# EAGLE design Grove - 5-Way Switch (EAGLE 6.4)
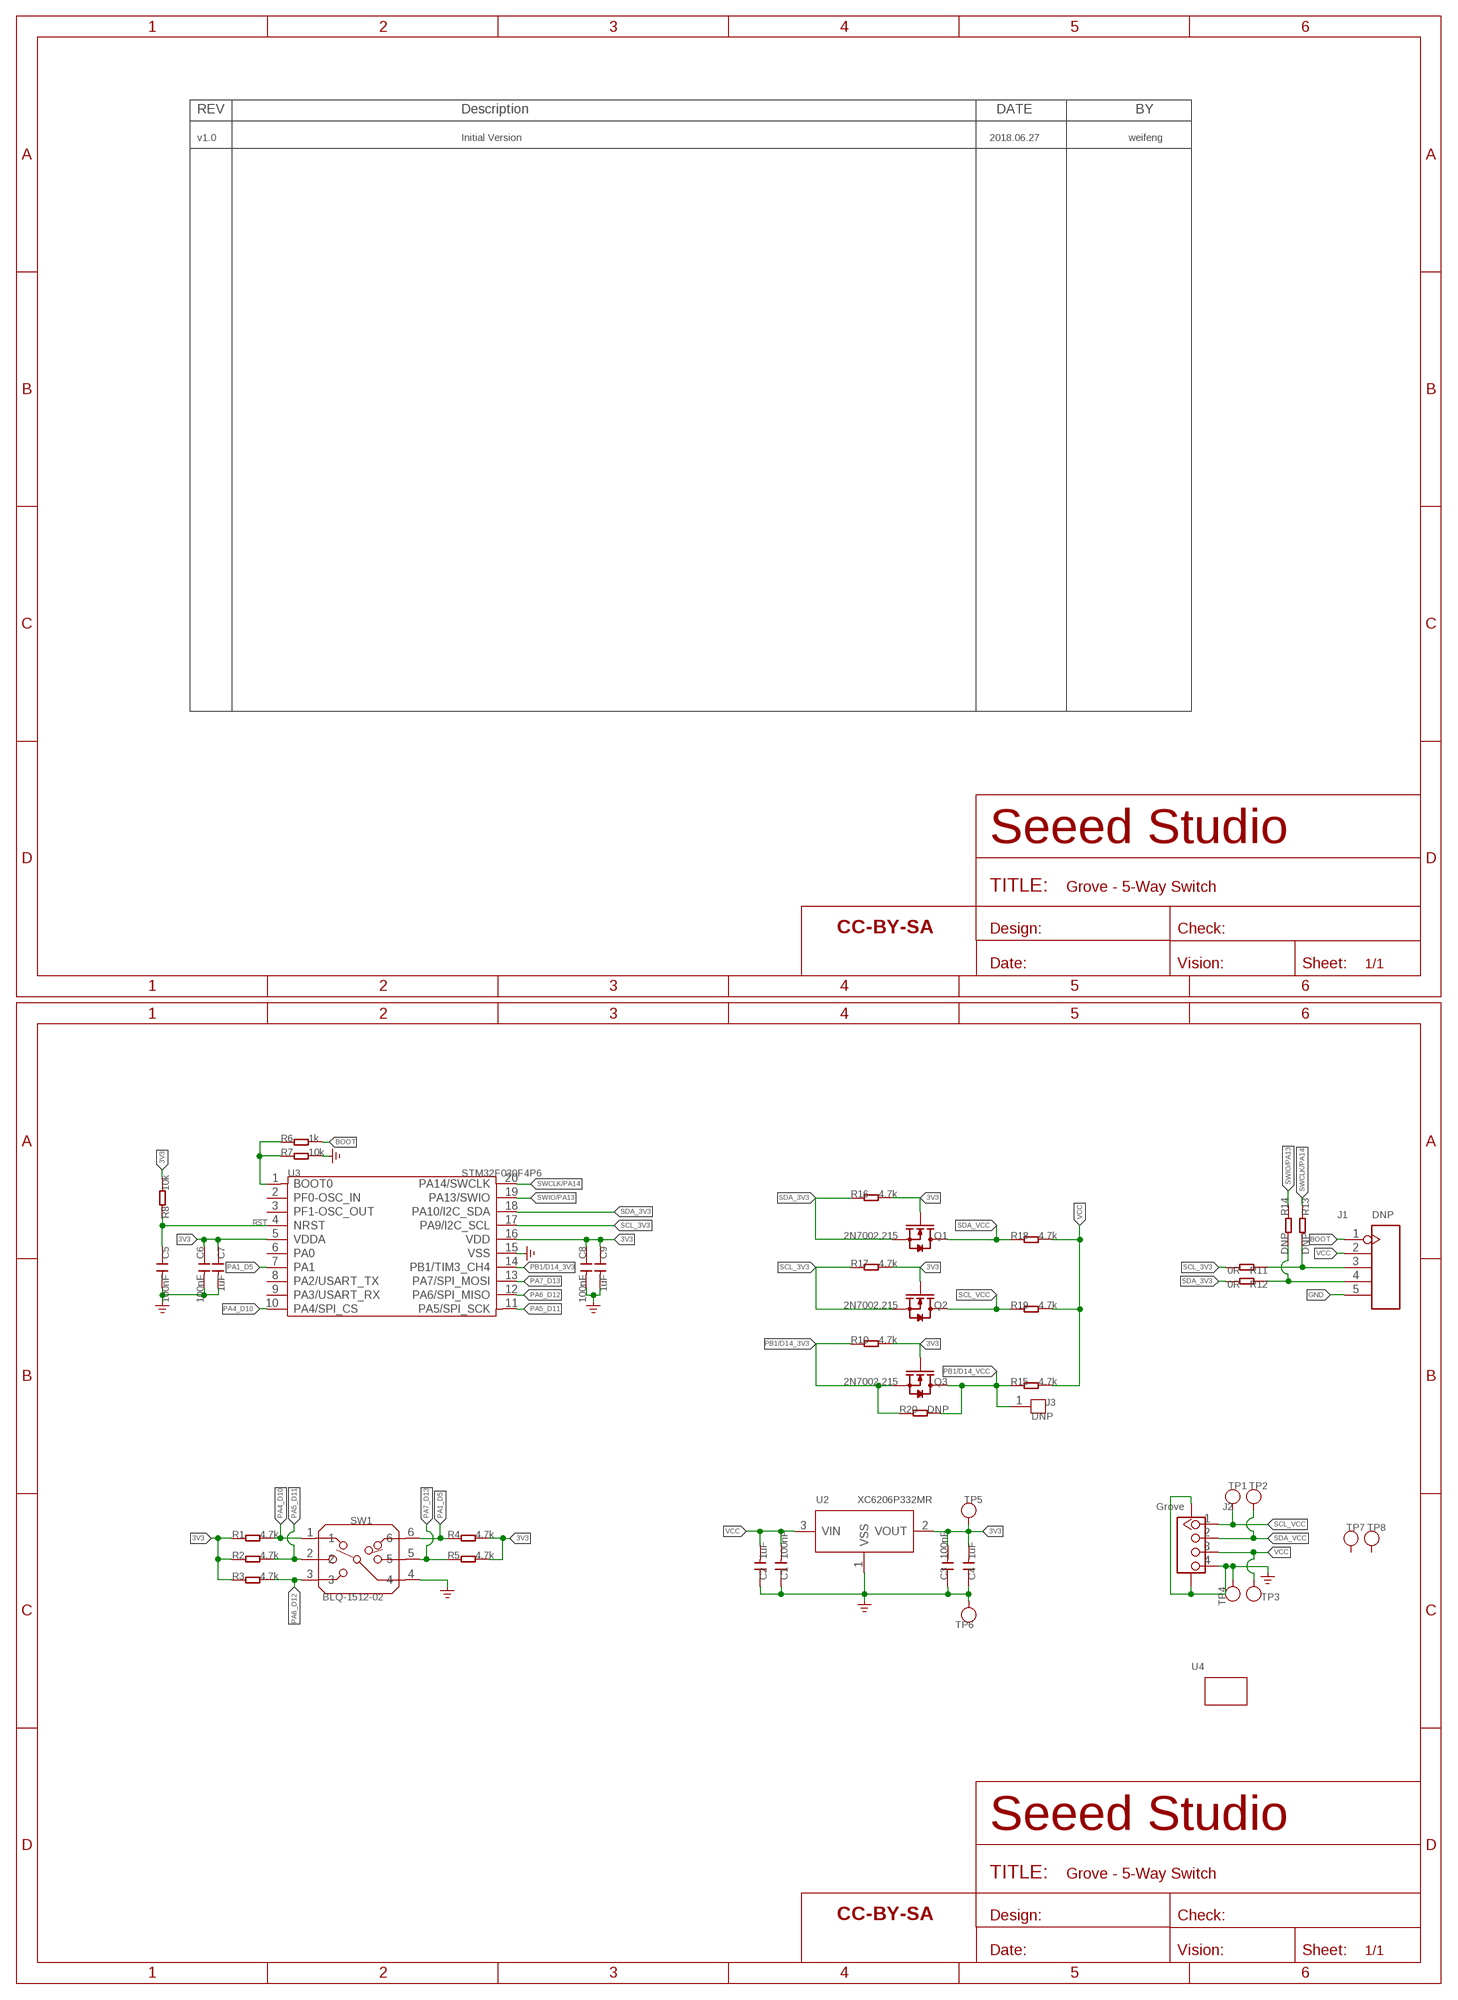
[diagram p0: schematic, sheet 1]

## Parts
C1  100nF  C-0603  [C0603]
C2  1uF  C-0603  [C0603]
C3  100nF  C-0603  [C0603]
C4  1uF  C-0603  [C0603]
C5  100nF  C-0603  [C0603]
C6  100nF  C-0603  [C0603]
C7  1uF  C-0603  [C0603]
C8  100nF  C-0603  [C0603]
C9  1uF  C-0603  [C0603]
FR1  SEEEDSTUDIO-OPEN-SCH-FRAME  [SEEEDSTUDIO-PCB-FRAME]
J1  DNP  HEADER-5P-SMD2.54  [H5-SMD-2.54]
J2  Grove  GROVE-CONNECTOR-SMD'DD'  [HW4-SMD-2.0]
J3  DNP  HEADER-1P-35  [1P-65/35MIL]
Q1  2N7002,215  MOSFET-N'SOT23'  [SOT-23]
Q2  2N7002,215  MOSFET-N'SOT23'  [SOT-23]
Q3  2N7002,215  MOSFET-N'SOT23'  [SOT-23]
R1  4.7k  R-0603  [R0603]
R2  4.7k  R-0603  [R0603]
R3  4.7k  R-0603  [R0603]
R4  4.7k  R-0603  [R0603]
R5  4.7k  R-0603  [R0603]
R6  1k  R-0603  [R0603]
R7  10k  R-0603  [R0603]
R8  10k  R-0603  [R0603]
R10  4.7k  R-0603  [R0603]
R11  0R  R-0603  [R0603]
R12  0R  R-0603  [R0603]
R13  DNP  R-0603  [R0603]
R14  DNP  R-0603  [R0603]
R15  4.7k  R-0603  [R0603]
R16  4.7k  R-0603  [R0603]
R17  4.7k  R-0603  [R0603]
R18  4.7k  R-0603  [R0603]
R19  4.7k  R-0603  [R0603]
R20  DNP  R-0603  [R0603]
SW1  BLQ-1512-02  SWITCH-6P  [SW6-3.25-10.2X10.2X6MM]
TP1  TEST-POINT'4545'  [TP-D45MIL]
TP2  TEST-POINT'4545'  [TP-D45MIL]
TP3  TEST-POINT'4545'  [TP-D45MIL]
TP4  TEST-POINT'4545'  [TP-D45MIL]
TP5  TEST-POINT'4545'  [TP-D45MIL]
TP6  TEST-POINT'4545'  [TP-D45MIL]
TP7  TEST-POINT'4545'  [TP-D45MIL]
TP8  TEST-POINT'4545'  [TP-D45MIL]
U2  XC6206P332MR  PMIC-XC6206PMR  [SOT-23]
U3  STM32F030F4P6  MCU-STM32F030  [TSSOP20-0.65-6.5X4.4MM]
U4  GROVE-TOP  [GROVE-1*2-TEST-PLATFORM-TOP]
U$4  SEEEDSTUDIO-OPEN-SCH-FRAME  [SEEEDSTUDIO-PCB-FRAME]

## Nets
3V3: C3.2 C4.2 C6.1 C7.1 C8.1 C9.1 Q1.1(G) Q2.1(G) Q3.1(G) R1.1 R2.1 R3.1 R4.2 R5.2 R8.2 R10.2 R16.2 R17.2 TP5.T U2.2(VOUT) U3.5(VDDA) U3.16(VDD)
!RST: C5.1 R8.1 U3.4(NRST)
BOOT: J1.1 R6.2
GND: C1.1 C2.1 C3.1 C4.1 C5.2 C6.2 C7.2 C8.2 C9.2 J1.5 J2.4 J2.SS1 J2.SS2 R7.2 SW1.4 TP4.T TP6.T U2.1(VSS) U3.15(VSS) ; supply symbol labelled GND_POWER
N$1: R6.1 R7.1 U3.1(BOOT0)
N$3: J1.3 R11.1 R13.2
N$4: J1.4 R12.1 R14.2
PA1_D5: R4.1 SW1.6 U3.7(PA1)
PA4_D10: R1.2 SW1.1 U3.10(PA4/SPI_CS)
PA5_D11: R2.2 SW1.2 U3.11(PA5/SPI_SCK)
PA6_D12: R3.2 SW1.3 U3.12(PA6/SPI_MISO)
PA7_D13: R5.1 SW1.5 U3.13(PA7/SPI_MOSI)
PB1/D14_3V3: Q3.2(S) R10.1 R20.1 U3.14(PB1/TIM3_CH4)
PB1/D14_VCC: J3.1 Q3.3(D) R15.1 R20.2
SCL_3V3: Q2.2(S) R11.2 R17.1 U3.17(PA9/I2C_SCL)
SCL_VCC: J2.1 Q2.3(D) R19.1 TP1.T
SDA_3V3: Q1.2(S) R12.2 R16.1 U3.18(PA10/I2C_SDA)
SDA_VCC: J2.2 Q1.3(D) R18.1 TP2.T
SWCLK/PA14: R13.1 U3.20(PA14/SWCLK)
SWIO/PA13: R14.1 U3.19(PA13/SWIO)
VCC: C1.2 C2.2 J1.2 J2.3 R15.2 R18.2 R19.2 TP3.T U2.3(VIN)
Unconnected: TP7.T TP8.T U3.2(PF0-OSC_IN) U3.3(PF1-OSC_OUT) U3.6(PA0) U3.8(PA2/USART_TX) U3.9(PA3/USART_RX)

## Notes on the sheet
- v1.0 | Initial Version | 2018.06.27 | weifeng

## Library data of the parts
C1-C9 = Discrete-small:C*: Ceramic Capacitors
FR1 U$4 = moudle-new:SEEEDSTUDIO-OPEN-SCH-FRAME
J1 = Connector-new:HEADER-5P
J2 = Connector-new:GROVE-CONNECTOR-SMD: 4P-SMD-2.0:320110030;4P-SMD-2.0-90D:320110032
J3 = Connector-new:HEADER-1P
Q1-Q3 = Discrete-new:MOSFET-N
R1-R8 R10-R20 = Discrete-small:R*
SW1 = Discrete-new:SWITCH-6P
TP1-TP8 = Discrete-new:TEST-POINT; PARTNO: DNP
U2 = IC-new:PMIC-XC6206P: LOW ESR Cap.Compatible Positive Voltage Regulators
U3 = IC-new:MCU-STM32F030
U4 = moudle-new:GROVE

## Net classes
3 usbvcc: width 0.203 mm, drill 0.305 mm, clearance 0.203 mm

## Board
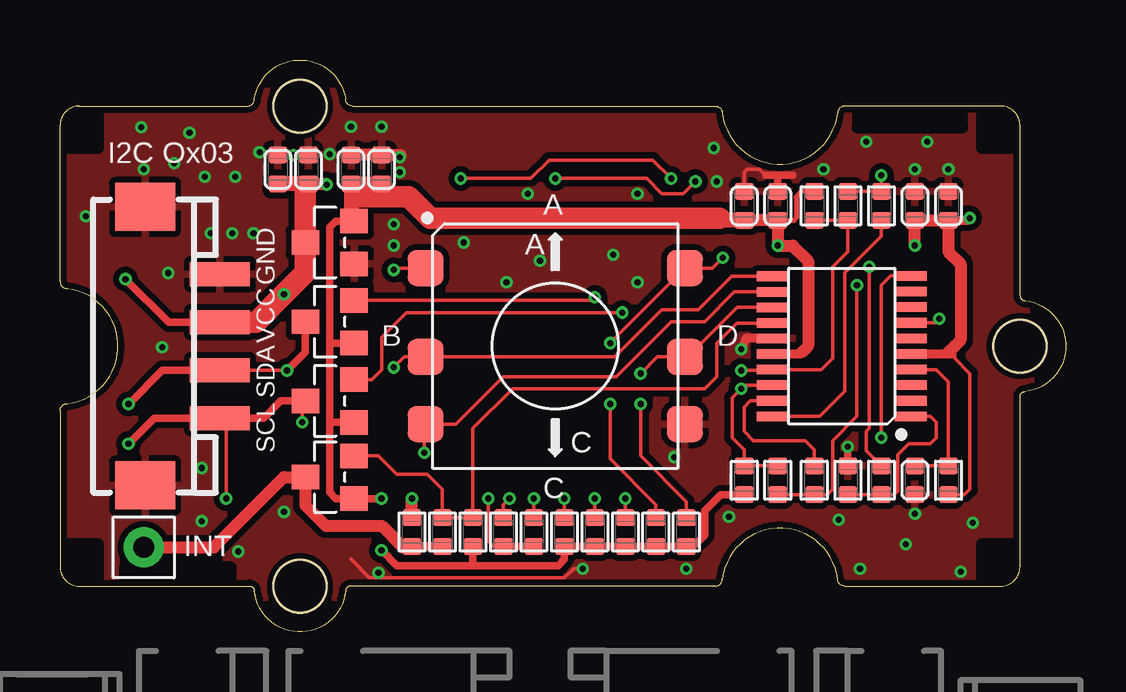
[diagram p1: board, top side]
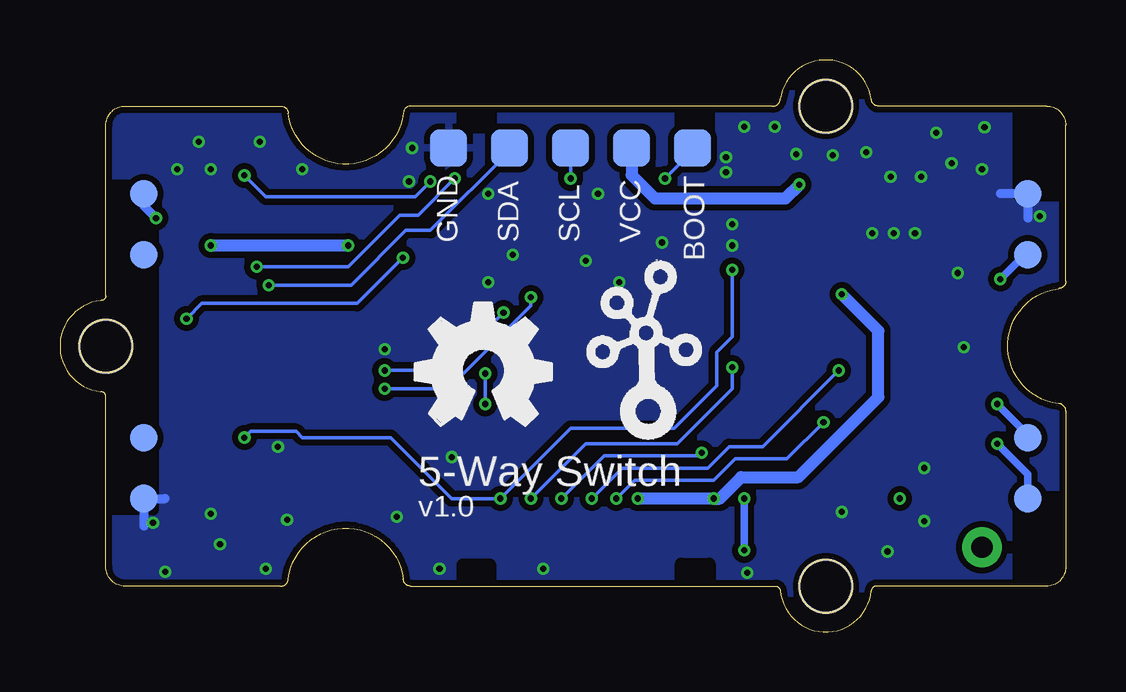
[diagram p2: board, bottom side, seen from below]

Size 41.91 x 23.83 mm. Coordinates in mm from the lower left corner, seen from the top.
Copper layers (1*16): Top 0.035mm / dielectric 1.5mm / Bottom 0.035mm
Design rules "SeeedStudio_2layer_DRU_no_angle_20140221": minimum track width 1mil, minimum drill 10mil, track to track 6mil, track to pad 6mil, pad to pad 6mil, via to via 6mil, smd to smd 0mil, copper to edge 10mil, drill to drill 10mil, minimum pad ring 4mil, minimum via ring 4mil, stop-mask expansion 2mil, vias tented up to drill 25mil, thermal gap 10mil

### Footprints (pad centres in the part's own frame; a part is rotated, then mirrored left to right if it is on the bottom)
C0603 = smd 0.762 x 0.696: 1 0,0.602; 2 0,-0.602
H5-SMD-2.54 = smd 1.524 x 1.524: 1 0,5.08; 2 0,2.54; 3 0,0; 4 0,-2.54; 5 0,-5.08
HW4-SMD-2.0 = smd 1 x 2.5: 1 -3,0; 2 -1,0; 3 1,0; 4 3,0 | smd 2 x 2.5: SS1 -5.8,3.123; SS2 5.8,3.123
1P-65/35MIL = drill 0.889 pad 1.651: 1 0,0
SOT-23 = smd 1.143 x 1.016: 1 1.016,-0.889; 2 1.016,0.889; 3 -1.016,0
R0603 = smd 0.762 x 0.696: 1 0,0.602; 2 0,-0.602
SW6-3.25-10.2X10.2X6MM = smd 1.5 x 1.5: 1 -5.4,3.25; 2 -5.4,-0.45; 3 -5.4,-3.25; 4 5.4,-3.25; 5 5.4,-0.45; 6 5.4,3.25
TP-D45MIL = smd 1.143 x 1.143: T 0,0
SOT-23' = smd 1.016 x 1.143: 1 -0.889,-1.016; 2 0.889,-1.016; 3 0,1.016
TSSOP20-0.65-6.5X4.4MM = smd 0.4 x 1.35: 1 -2.925,-2.875; 2 -2.275,-2.875; 3 -1.625,-2.875; 4 -0.975,-2.875; 5 -0.325,-2.875; 6 0.325,-2.875; 7 0.975,-2.875; 8 1.625,-2.875; 9 2.275,-2.875; 10 2.925,-2.875; 11 2.91,2.875; 12 2.26,2.875; 13 1.61,2.875; 14 0.96,2.875; 15 0.325,2.875; 16 -0.325,2.875; 17 -0.975,2.875; 18 -1.625,2.875; 19 -2.275,2.875; 20 -2.925,2.875
GROVE-1*2-TEST-PLATFORM-TOP = hole 2.2: 10.635,10; 10.635,-10; -19.365,0

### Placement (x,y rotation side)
C1  9.08,19.27 0 top
C2  10.35,19.27 0 top
C3  13.4,19.27 0 top
C4  12.13,19.27 0 top
C5  35.62,6.32 0 top
C6  35.62,17.75 180 top
C7  37.02,17.75 180 top
C8  29.91,17.75 180 top
C9  28.51,17.75 180 top
FR1  not placed on the board
J1  20.64,20.16 270 bottom
J2  6.67,11.91 90 top
J3  3.49,3.53 0 top
Q1  11.24,12.92 0 top
Q2  11.24,9.62 0 top
Q3  11.24,6.45 0 top
R1  23.56,4.16 180 top
R2  22.29,4.16 180 top
R3  21.02,4.16 180 top
R4  24.83,4.16 0 top
R5  26.1,4.16 0 top
R6  34.22,6.32 180 top
R7  32.83,6.32 180 top
R8  37.02,6.32 0 top
R10  17.21,4.16 0 top
R11  32.83,17.75 0 top
R12  29.91,6.32 180 top
R13  34.22,17.75 180 top
R14  31.43,6.32 0 top
R15  14.67,4.16 180 top
R16  28.51,6.32 0 top
R17  31.43,17.75 180 top
R18  19.75,4.16 0 top
R19  18.48,4.16 0 top
R20  15.94,4.16 0 top
SW1  20.64,11.91 0 top
TP1  1.59,5.56 0 bottom
TP2  1.59,8.1 0 bottom
TP3  1.59,15.72 0 bottom
TP4  1.59,18.26 0 bottom
TP5  38.42,18.26 0 bottom
TP6  38.42,5.56 0 bottom
TP7  38.42,15.72 0 bottom
TP8  38.42,8.1 0 bottom
U2  XC6206P332MR  [SOT-23']  11.24,16.23 90 top
U3  32.57,11.91 90 top
U4  20.64,11.91 180 top
U$4  not placed on the board
U$5  [OSHW_FILLX200_NOTEXT]  27.11,8.61 0 bottom
U$7  [TWIGLOGO]  17.46,8.99 0 bottom

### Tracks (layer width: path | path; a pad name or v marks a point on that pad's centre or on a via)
3V3  (via drill 0.25 pad 0.51)
  Top 0.152: 37.02,11.58 35.78,11.58 U3.5 | R8.2 37.69,5.72 37.91,5.94 37.91,10.77 37.27,11.4 | 37.27,11.4 37.02,11.65 37.02,11.64 37.07,11.58 | 37.27,11.91 37.27,11.4
  Top 0.203: C8.1 30.57,17.15 30.67,17.24 30.67,18.13 30.89,18.35 R17.2
  Top 0.305: U2.2 11.49,17.12 11.24,16.86 11.24,12.04 | 11.24,12.04 11.24,8.73 | 11.24,8.73 11.24,5.81 11.49,5.56 Q3.1 v13.4,5.56 | Q2.1 11.24,8.73 | Q1.1 11.24,12.04 | R16.2 27.53,5.72 26.86,5.05 26.86,4.03 26.38,3.56 R5.2 R4.2 R1.1 R2.1 R3.1 21.02,3.02 20.76,2.76 17.21,2.76 | 17.21,2.76 14.03,2.76 v13.4,3.4 | R10.2 17.21,2.76
  Top 0.381: 35.78,11.58 37.07,11.58 37.15,11.65 | U3.16 30.85,11.58 30.92,11.65 | C7.1 37.81,17.15 v37.91,17.24
  Top 0.508: v35.62,16.1 C6.1 C7.1 37.02,15.85 37.53,15.34 37.53,12.16 37.27,11.91 37.02,11.65 | C9.1 C8.1 v29.91,16.1 30.54,16.1 31.18,15.46 31.18,11.91 30.92,11.65 | 12.38,18.13 12.38,18.39 12.13,18.64
  Top 0.635: U2.2 12.13,17.24 12.13,18.64 C4.2 C3.2 | C9.1 27.59,17.15 27.49,17.24
  Top 0.889: 27.49,17.24 15.43,17.24 14.54,18.13 12.38,18.13
  Bottom 0.305: v13.4,3.4 v13.4,5.56
  Bottom 0.381: TP5.T 38.42,17.75 v37.91,17.24
  Bottom 0.508: v29.91,16.1 v35.62,16.1
!RST
  Top 0.152: C5.1 R8.1 37.02,10.43 36.51,10.93 U3.4
BOOT  (via drill 0.25 pad 0.51)
  Top 0.152: v33.72,15.21 33.72,8.48 33.59,8.35 33.59,7.56 R6.2 | v16.7,18.89 19.62,18.89 20.38,19.66 24.7,19.66 v25.46,18.89
  Bottom 0.152: v33.72,15.21 29.91,15.21 27.75,17.37 26.98,17.37 v25.46,18.89 | v16.7,18.89 15.71,19.88 15.71,20.01 J1.1
GND  (via drill 0.25 pad 0.51)
  Top 0.152: v21.78,2.64 21.4,2.64 21.02,2.26 12.89,2.26 12.13,3.02 | C9.2 28.51,19.15 28.64,19.27 29.14,19.27 29.4,19.02
  Top 0.305: R7.2 v32.83,7.72 | 29.4,19.02 29.91,19.02 | 29.91,19.02 30.54,19.02 | C8.2 29.91,19.02
  Top 0.381: U3.15 28.58,12.23 v28.38,11.78
  Top 0.508: C4.1 C3.1 14.19,19.88 v14.16,19.78
  Bottom 0.381: 38.42,4.42 TP6.T 37.53,5.56 | 1.59,17.24 TP4.T 2.73,18.26
  other vias: 13.9,16.1 3.49,19.27 4.76,19.53 5.4,20.8 3.39,21.03 1.08,17.32 4.25,11.86 9.71,19.86 35.62,4.92 27.37,18.77 35.62,19.27 37.02,19.27 5.9,6.83 5.9,4.62 13.9,16.99 14.16,19.15 4.51,14.96 16.83,16.23 24.06,14.58 18.6,14.58 23.05,15.72 32.45,4.67 33.34,2.64 37.53,2.51 38.03,4.54 27.87,4.8 26.1,2.64 6.28,16.61 7.17,16.61 8.06,16.61 25.59,7.29 8.32,19.99 6.03,18.97 7.3,18.97 19.49,18.26 24.06,18.26 27.24,20.16 12.13,21.05 13.4,21.05 11.24,19.91 7.43,3.35 9.33,5 13.27,2.46 31.81,19.27 33.59,20.42 36.13,20.42 35.24,3.65 20,15.46
  pour Top (isolate 0.254): -0.95,23.85 41.59,23.85 41.59,-0.28 -0.95,-0.28
  pour Bottom (isolate 0.254): -0.95,23.85 41.59,23.85 41.59,-0.28 -0.95,-0.28
N$1
  Top 0.152: R7.1 R6.1 34.77,5.72 34.91,5.86 34.91,7.39 35.37,7.84 36.26,7.84 36.51,8.1 36.51,8.73 36.26,8.98 U3.1
N$3  (via drill 0.25 pad 0.51)
  Top 0.152: R11.1 R13.2 v34.22,19.02 | v20.64,18.89 24.45,18.89 25.08,18.26 25.97,18.26 v26.48,18.77
  Bottom 0.152: v26.48,18.77 27.11,18.13 33.34,18.13 v34.22,19.02 | J1.3 v20.64,18.89
N$4  (via drill 0.25 pad 0.51)
  Top 0.152: R12.1 R14.2 31.97,5.72 32.19,5.94 32.19,7.97 33.21,8.99 v33.21,14.45
  Bottom 0.152: v33.21,14.45 29.78,14.45 27.49,16.73 26.48,16.73 23.18,20.04 J1.4
PA1_D5  (via drill 0.25 pad 0.51)
  Top 0.152: U3.7 36.6,12.88 v36.64,13.05 | R4.1 24.83,5.3 22.92,7.21 v22.92,9.5 | v22.92,12.04 22.91,12.04 SW1.6 27.19,15.16 v27.62,15.59
  Bottom 0.152: v22.92,9.5 v22.92,12.04 | v27.62,15.59 29.53,13.69 36,13.69 v36.64,13.05
PA4_D10  (via drill 0.25 pad 0.51)
  Top 0.152: R1.2 v23.56,5.56 | SW1.1 13.98,15.16 v13.9,15.08 | U3.10 34.61,14.83 34.22,14.45 v34.22,8.1
  Bottom 0.152: v13.9,15.08 13.9,12.29 14.54,11.65 14.54,10.26 16.32,8.48 20.64,8.48 v23.56,5.56 25.59,5.56 28.13,8.1 31.81,8.1 32.06,8.35 33.97,8.35 v34.22,8.1
PA5_D11  (via drill 0.25 pad 0.51)
  Top 0.152: U3.11 27.99,14.82 26.6,13.43 25.08,13.43 23.11,11.46 SW1.2 14.34,11.46 v13.9,11.02 | R2.2 v22.29,5.56
  Bottom 0.152: v22.29,5.56 20,7.84 16.19,7.84 13.9,10.13 v13.9,11.02
PA6_D12  (via drill 0.25 pad 0.51)
  Top 0.152: U3.12 28.1,14.17 26.86,12.92 25.46,12.92 23.18,10.64 18.48,10.64 16.5,8.66 SW1.3 15.17,8.66 v15.17,7.46 | R3.2 v21.02,5.56
  Bottom 0.152: v21.02,5.56 19.24,7.34 15.3,7.34 v15.17,7.46
PA7_D13  (via drill 0.25 pad 0.51)
  Top 0.152: U3.13 28.21,13.52 26.15,11.46 SW1.5 24.88,11.46 v24.19,10.77 | R5.1 26.1,5.43 24.19,7.34 v24.19,9.5
  Bottom 0.152: v24.19,9.5 v24.19,10.77
PB1/D14_3V3
  Top 0.152: R10.1 17.17,4.76 | U3.14 28.2,12.87 27.37,12.04 27.37,10.64 26.86,10.13 18.86,10.13 17.21,8.48 17.21,4.8 17.17,4.76 | Q3.2 13.27,7.34 14.03,6.57 15.3,6.57 15.94,5.94 R20.1 17.17,4.76
PB1/D14_VCC
  Top 0.381: R15.1 R20.2
  Top 0.508: J3.1 6.41,3.53 9.33,6.45 Q3.3 10.22,5.27 11.07,4.42 13.4,4.42 14.29,3.53 14.63,3.53 R15.1
SCL_3V3  (via drill 0.25 pad 0.51)
  Top 0.152: Q2.2 12.99,10.51 13.4,10.91 13.4,12.28 14.42,13.31 v23.43,13.31 | v28.38,10.89 29.66,10.89 U3.17 31.73,10.93 32.19,11.4 32.19,15.21 32.83,15.85 R11.2 R17.1 | R17.1 31.34,17.15 31.3,17.12 31.4,17.12 R17.1
  Bottom 0.152: v23.43,13.31 25.84,10.89 v28.38,10.89
SCL_VCC  (via drill 0.25 pad 0.51)
  Top 0.152: v6.92,5.56 6.92,8.91 | R19.1 18.48,5.3 v18.73,5.56 | v10.09,8.73 10.09,9.62
  Top 0.305: Q2.3 10.09,9.62 9.21,9.62 8.49,8.91 6.92,8.91 J2.1 3.92,8.91 v2.86,7.84
  Bottom 0.152: v18.73,5.56 17.97,6.32 14.67,6.32 13.78,7.21 11.62,7.21 v10.09,8.73
  Bottom 0.305: v2.86,7.84 1.59,6.57 TP1.T
SDA_3V3  (via drill 0.25 pad 0.51)
  Top 0.152: Q1.2 22.16,13.81 v22.29,13.94 | U3.18 28.54,10.28 v28.38,10.13 28,9.75 28,8.1 28.51,7.59 R16.1 R12.2
  Bottom 0.152: v28.38,10.13 25.74,10.13 22.29,13.59 v22.29,13.94
SDA_VCC  (via drill 0.25 pad 0.51)
  Top 0.152: R18.1 v19.75,5.56 | v9.46,10.89 6.68,10.89 J2.2
  Top 0.305: J2.2 4.27,10.91 v2.86,9.5 | v9.46,10.89 10.22,11.65 Q1.3
  Bottom 0.152: v19.75,5.56 18.48,6.83 14.92,6.83 14.03,7.72 12.63,7.72 v9.46,10.89
  Bottom 0.305: TP2.T 1.59,8.23 v2.86,9.5
SWCLK/PA14
  Top 0.152: U3.20 31.65,8.98 32.7,10.03 32.7,14.96 34.22,16.48 R13.1
SWIO/PA13
  Top 0.152: R14.1 31.43,7.59 31.05,7.97 28.89,7.97 28.51,8.35 28.51,9.37 28.7,9.56 28.76,9.62 28.77,9.63 U3.19
VCC  (via drill 0.25 pad 0.51)
  Top 0.152: R19.2 18.06,3.56 17.84,3.78 v17.84,5.56
  Top 0.305: J2.3 4.52,12.91 v2.73,14.7 | R19.2 R18.2
  Top 0.508: C2.2 11.08,18.67 v11.11,18.64 | R15.2 v14.67,5.56
  Top 0.635: 10.22,18.51 10.22,18.55 C2.2 C1.2
  Top 0.889: 10.22,18.51 U2.3 10.22,14.96 v9.33,14.07 8.17,12.91 J2.3
  Bottom 0.152: v14.67,5.56 14.54,5.56
  Bottom 0.305: TP3.T 1.71,15.72 v2.73,14.7
  Bottom 0.508: v17.84,5.56 v14.67,5.56 14.41,5.56 13.52,6.45 11.14,6.45 7.81,9.78 7.81,12.54 v9.33,14.07 | J1.2 18.1,19.04 17.12,18.06 11.69,18.06 v11.11,18.64

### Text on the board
tPlace: I2C Ox03 | A | GND | VCC | B | D | SDA | SCL | C | INT
bPlace: BOOT | VCC | SCL | SDA | GND | 5-Way Switch | v1.0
